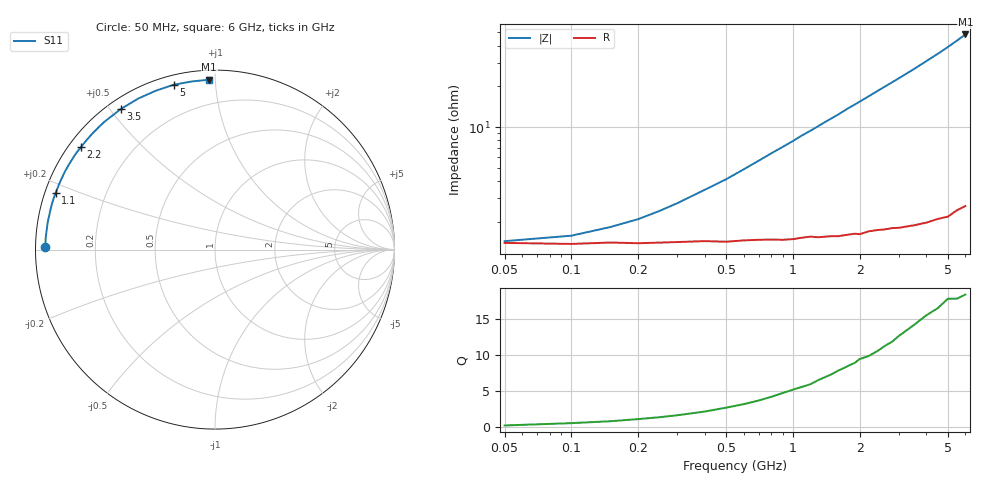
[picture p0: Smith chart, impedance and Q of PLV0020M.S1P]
! Infineon Technologies  Discrete & RF Semiconductors
! BAR 64-04W /-05W /-06W
! Si PIN Diode in SOT323
! IF = 20 mA
! S-Parameters:  October  2008
# GHz  S  MA  R  50
!  f  S11
! GHz  MAG  ANG
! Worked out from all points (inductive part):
!   34 points, 50 MHz to 6 GHz, reference 50 ohm
!   read as one part to ground: L = 1.24 nH near 600 MHz
!   highest Q = 18.3 at 6 GHz (marker M1), where L = 1.28 nH
!   S11 on the Smith chart (normalised r, x): 50 MHz: 0.03, +0.01; 1.1 GHz: 0.03, +0.17; 2.2 GHz: 0.03, +0.34; 3.5 GHz: 0.04, +0.53; 5 GHz: 0.04, +0.78; 6 GHz: 0.05, +0.96
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0.05  0.9453 179.2
0.1  0.9462 178.2
0.15  0.945 177.3
0.2  0.9456 176.4
0.4  0.9439 172.8
0.5  0.9445 171.1
0.8  0.9431 165.7
0.9  0.9435 164.0
1  0.9431 162.3
1.1  0.942 160.5
1.2  0.9413 158.9
1.3  0.9422 157.2
1.4  0.942 155.5
1.6  0.9423 152.3
1.8  0.9415 148.9
1.9  0.9412 147.4
2  0.9421 145.8
2.2  0.9404 142.7
2.4  0.9402 139.6
2.6  0.9407 136.6
2.8  0.9407 133.7
3  0.9417 130.8
3.5  0.9427 123.8
4  0.944 116.9
4.5  0.9446 110.4
5  0.9468 104.1
5.5  0.9458 97.9
6  0.9469 92.0
